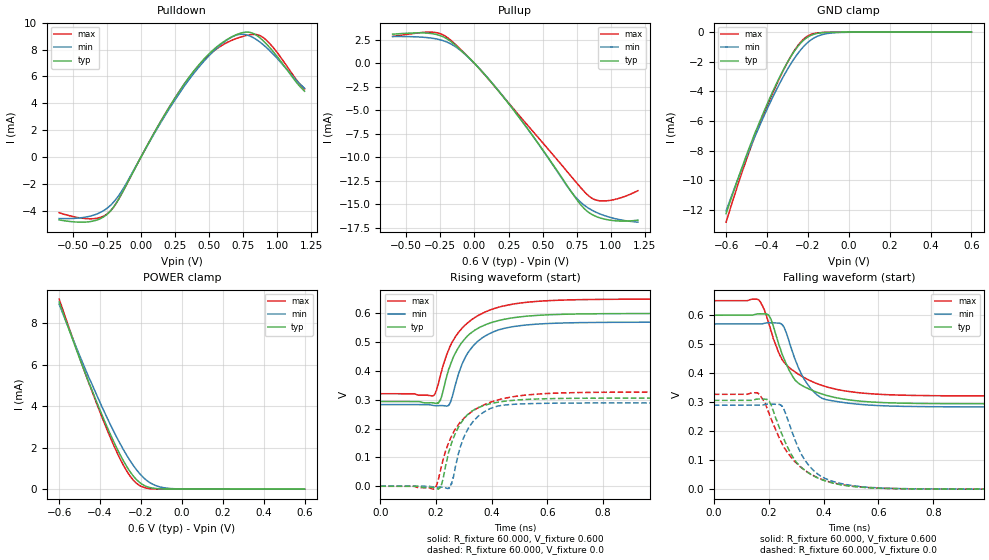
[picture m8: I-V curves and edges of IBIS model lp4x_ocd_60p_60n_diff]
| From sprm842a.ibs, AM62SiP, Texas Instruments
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|   Model lp4x_ocd_60p_60n_diff
[Model] lp4x_ocd_60p_60n_diff
Model_type I/O
Polarity   Non-Inverting
Enable   Active-High
Vinl =  0.0V
Vinh =  0.900V
Vmeas =  0.600V
C_comp   2.191pF   1.975pF   2.458pF
[Model Spec]
Vinh   0.900V   0.900V   0.900V
Vinl   0.0V   0.0V   0.0V
Vmeas   0.600V   NA   NA
[Temperature Range]   25.000   0.125k   -40.000
[Voltage Range]   0.600V   0.570V   0.650V
[Pullup Reference]   0.600V   0.570V   0.650V
[Pulldown Reference]   0.0V   0.0V   0.0V
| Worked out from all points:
|   slope of the pulldown table from 0 to 0.09 V, typ, clamps not added: 53.7 ohm
|   slope of the pullup table from 0 to 0.09 V, typ, clamps not added: 62.7 ohm
|   GND clamp passes 1 mA (typ) near -0.25 V on its own axis
|   POWER clamp passes 1 mA (typ) near -0.26 V on its own axis
|   rising waveform, R_fixture 60.000, V_fixture 0.600: 20-80 % time 104ps typ, 95.8ps min, 121ps max; typ from 0.294 V to 0.6 V
|   rising waveform, R_fixture 60.000, V_fixture 0.0: 20-80 % time 77.7ps typ, 72.1ps min, 114ps max; typ from 0 V to 0.306 V
|   falling waveform, R_fixture 60.000, V_fixture 0.600: 20-80 % time 101ps typ, 85.7ps min, 129ps max; typ from 0.6 V to 0.294 V
|   falling waveform, R_fixture 60.000, V_fixture 0.0: 20-80 % time 111ps typ, 98.4ps min, 130ps max; typ from 0.306 V to 0 V
[Pulldown]
|Voltage   I(typ)   I(min)   I(max)
-600mV    -4.672mA   -4.571mA   -4.137mA
-354mV    -4.766mA   -4.339mA   -4.584mA
-221mV    -3.975mA   -3.563mA   -3.979mA
-126mV    -2.436mA   -2.275mA   -2.428mA
120mV     2.217mA    2.136mA    2.211mA
328mV     5.591mA    5.421mA    5.575mA
499mV     7.678mA    7.538mA    7.592mA
669mV     8.962mA    8.947mA    8.701mA
783mV     9.299mA    9.068mA    9.069mA
897mV     8.653mA    8.357mA    8.892mA
973mV     7.809mA    7.626mA    8.115mA
1.2V      4.9mA      5.117mA    5.072mA
[Pullup]
|Voltage   I(typ)   I(min)   I(max)
-600mV    3.099mA    2.851mA    2.858mA
-278mV    3.066mA    2.591mA    3.26mA
-202mV    2.61mA     2.263mA    2.778mA
-107mV    1.503mA    1.424mA    1.564mA
44.21mV   -687uA     -680.9uA   -702.8uA
234mV     -3.978mA   -3.946mA   -3.927mA
461mV     -8.382mA   -8.395mA   -7.778mA
707mV     -13.59mA   -13.6mA    -11.98mA
840mV     -15.87mA   -15.43mA   -14.12mA
897mV     -16.31mA   -15.87mA   -14.56mA
973mV     -16.62mA   -16.28mA   -14.62mA
1.2V      -16.68mA   -16.89mA   -13.54mA
[GND_clamp]
|Voltage   I(typ)   I(min)   I(max)
-600mV    -12.26mA   -12.07mA   -12.83mA
-535mV    -9.631mA   -9.657mA   -9.999mA
-483mV    -7.674mA   -7.84mA    -7.926mA
-457mV    -6.749mA   -6.974mA   -6.957mA
-378mV    -4.198mA   -4.571mA   -4.306mA
-326mV    -2.706mA   -3.156mA   -2.747mA
-287mV    -1.735mA   -2.22mA    -1.722mA
-248mV    -949.8uA   -1.424mA   -887.8uA
-209mV    -414uA     -806.6uA   -336.6uA
-157mV    -95.47uA   -302uA     -61.63uA
-78.26mV  -9.128uA   -53.02uA   -8.176uA
600mV     0A         0A         0A
[POWER_clamp]
|Voltage   I(typ)   I(min)   I(max)
-600mV    9.037mA    8.928mA    9.175mA
-457mV    5.197mA    5.441mA    5.165mA
-352mV    2.698mA    3.164mA    2.544mA
-313mV    1.878mA    2.4mA      1.683mA
-274mV    1.164mA    1.707mA    946.6uA
-248mV    770.3uA    1.297mA    560.2uA
-222mV    461.7uA    938.4uA    283.8uA
-196mV    245.9uA    638.8uA    120.5uA
-157mV    79.3uA     316.3uA    23.58uA
-117mV    22.65uA    136.3uA    6.083uA
-78.26mV  6.707uA    54.45uA    1.89uA
600mV     0A         0A         0A
[Ramp]
| variable   typ   min   max
dV/dt_r   0.184/76.987p   0.173/71.759p   0.196/0.114n
dV/dt_f   0.184/0.101n   0.172/85.547p   0.197/0.128n
R_load = 60.000
[Rising Waveform]
R_fixture= 60.000
V_fixture= 0.600
V_fixture_min= 0.570
V_fixture_max= 0.650
|time   V(typ)   V(min)   V(max)
0s        294.3mV    283.7mV    321.4mV
191ps     289.5mV    280.4mV    314.9mV
215ps     297mV      280.2mV    382.6mV
244ps     401.3mV    279.7mV    470.8mV
252ps     423.5mV    291.3mV    488.8mV
293ps     499.2mV    422.9mV    548.2mV
335ps     538.9mV    489.2mV    583mV
416ps     573.1mV    540.2mV    619.2mV
520ps     590.1mV    559.6mV    638.2mV
3ns       600mV      569.8mV    650mV
[Rising Waveform]
R_fixture= 60.000
V_fixture= 0.0
V_fixture_min= 0.0
V_fixture_max= 0.0
|time   V(typ)   V(min)   V(max)
0s        66.43uV    359.5uV    63.41uV
194ps     -5.305mV   -3.305mV   -9.078mV
219ps     3.233mV    -2.688mV   67.81mV
247ps     123.5mV    -7.544mV   154.5mV
256ps     151mV      8.355mV    174.2mV
297ps     229.7mV    164.1mV    232.2mV
333ps     263.3mV    224.9mV    262.1mV
401ps     288mV      272.4mV    293.6mV
509ps     300.7mV    286.1mV    315.3mV
3ns       306.2mV    289.5mV    327.1mV
[Falling Waveform]
R_fixture= 60.000
V_fixture= 0.600
V_fixture_min= 0.570
V_fixture_max= 0.650
|time   V(typ)   V(min)   V(max)
0s        600mV      569.8mV    650mV
163ps     604.9mV    569.8mV    653.3mV
203ps     595.5mV    573.9mV    562.3mV
242ps     486.2mV    572.2mV    459.6mV
260ps     440.6mV    550mV      433.4mV
296ps     376.2mV    448.2mV    404.2mV
360ps     340.1mV    340.2mV    370.1mV
405ps     325mV      309.8mV    354.6mV
520ps     304.8mV    293.5mV    333.5mV
3ns       294.3mV    283.7mV    321.3mV
[Falling Waveform]
R_fixture= 60.000
V_fixture= 0.0
V_fixture_min= 0.0
V_fixture_max= 0.0
|time   V(typ)   V(min)   V(max)
0s        306.2mV    289.5mV    327.1mV
161ps     310.9mV    289.5mV    331.5mV
202ps     303mV      293.4mV    258.7mV
244ps     199.9mV    290.8mV    165.8mV
258ps     166.8mV    270.5mV    141.3mV
300ps     93.62mV    160.7mV    90.84mV
347ps     54.92mV    80.95mV    55.26mV
405ps     28.85mV    37.22mV    29.86mV
505ps     9.498mV    12.36mV    10.39mV
3ns       64.37uV    355.4uV    62.76uV
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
